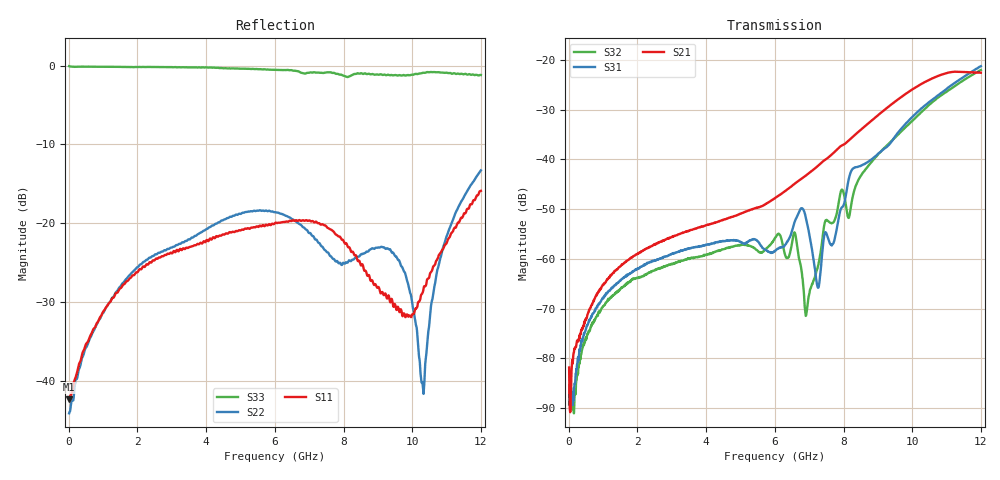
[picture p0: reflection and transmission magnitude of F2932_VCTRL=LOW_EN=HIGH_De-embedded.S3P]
! Integrated Device Technology
! Corporate Headquarters
! 6024 Silver Creek Valley Road
! San Jose, CA 95138  USA
! Phone:  1-408-284-8200
! Toll Free:  1-800-223-1366
! Webpage:  http://www.idt.com/
! Timing and RF Division
! 515 Groton Road, Suite 102
! Westford, MA 01886-6024
! Device:  F2932
! Description: High Reliability SP2T RF Switch
! Frequency:  0.05 -  8.00 GHz
! Package:  4x4 mm QFN Plastic Package: 16 pin
! Ports:  3 RF, 3 DC
!  Pin  1  = VDD
!  Pin  2  = VCTL
!  Pin  3  = RFC  =  Port 3
!  Pin  4  = GND
!  Pin  5  = EN
!  Pin  6  = GND
!  Pin  7  = GND
!  Pin  8  = GND
!  Pin  9  = RF1  =  Port 1
!  Pin 10  = GND
!  Pin 11  = GND
!  Pin  9  = RF2  =  Port 2
!  Pin 13  = GND
!  Pin 14  = GND
!  Pin 15  = GND
!  Pin 16  = NC
! State:  All Off
! VCTRL:  +0.00 Volts (Logic Low)
! EN:  +2.60 Volts (Logic High)
! Voltage:  +5.00 Volts
! Current:  0.412 mA
! Data:  The device was measured on a F2932 evaluation board which has
!  individual transmission lines to the RF pins.  Data was collected
!  using a calibrated network analyzer.  The evaluation board was
!  de-embedded using AFR (Keysight) technique.
!  The reference plane is the edge of the package pin.
! Misc:
!  Action Tracker AT0443
! Date Measured:  2018-10-10
! Date:  2018-10-11  MJV
! Note:
!  Integrated Device Technology supplies this data as a sample of measured
!  data at the package pin for this product.  Your particular data for this
!  product may vary.
!  Data was taken at 25 degrees C.
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# Hz S dB R 50
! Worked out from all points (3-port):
!   1200 points, 10 MHz to 12 GHz, reference 50 ohm
!   strongest paths, dB at 10 MHz, 3.01 GHz, 6.01 GHz, 9.01 GHz, 12 GHz:
!     S21: -81.8, -55.5, -47.8, -31.1, -22.6
!     S31: -88.4, -58.9, -58.4, -38.9, -21.3
!     S32: -89.3, -61.1, -55.8, -39.0, -22.0
!   lowest |S11| = -42.4 dB at 10 MHz (marker M1), VSWR 1.02, Z = 49.2 - j0.00123 ohm
!   |S11| at or under -10 dB: start of sweep to end of sweep
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1e7  -42.37 -179.9  -83.25 -1.6  -88.34 28.2
     -81.85 5.2  -44.15 179.0  -89.43 29.8
     -88.43 41.8  -89.27 32.8  -0.07 -0.4
2.28e9  -25.23 50.0  -57.86 87.3  -60.98 74.9
        -57.85 87.1  -24.64 44.2  -63.00 77.9
        -60.80 75.1  -62.99 77.5  -0.17 -45.2
6.01e9  -19.95 -8.3  -47.75 112.7  -58.44 75.9
        -47.76 113.0  -18.60 8.0  -55.78 78.2
        -58.43 77.2  -55.75 78.4  -0.54 -126.0
6.59e9  -19.69 -16.6  -44.82 118.5  -52.33 95.2
        -44.82 118.8  -19.71 4.3  -54.80 60.9
        -52.29 96.1  -54.86 61.1  -0.65 -139.2
6.92e9  -19.63 -20.4  -43.16 119.9  -52.29 33.0
        -43.17 120.1  -20.83 -0.8  -71.31 101.9
        -52.21 33.1  -71.03 99.8  -0.95 -143.7
7.26e9  -20.02 -24.2  -41.26 121.1  -65.94 -55.4
        -41.26 121.3  -22.44 -9.5  -61.46 172.4
        -65.82 -53.9  -61.35 171.6  -0.87 -149.6
8.23e9  -23.67 -42.6  -35.71 116.2  -42.25 -179.2
        -35.72 116.5  -24.76 -65.1  -48.93 178.2
        -42.26 -179.2  -48.91 178.1  -1.26 -165.3
9.58e9  -30.61 -133.7  -27.98 89.0  -34.68 140.7
        -27.98 89.3  -24.64 -105.2  -35.10 139.8
        -34.67 140.8  -35.08 139.8  -1.25 154.0
1.03e10  -28.85 136.2  -24.70 64.4  -29.59 115.5
         -24.70 64.7  -40.20 177.4  -30.34 119.2
         -29.58 116.0  -30.31 119.2  -0.92 138.8
1.2e10  -15.90 92.7  -22.57 0.3  -21.24 48.8
        -22.58 0.7  -13.30 84.8  -22.05 53.8
        -21.26 49.2  -22.04 53.8  -1.18 109.2
